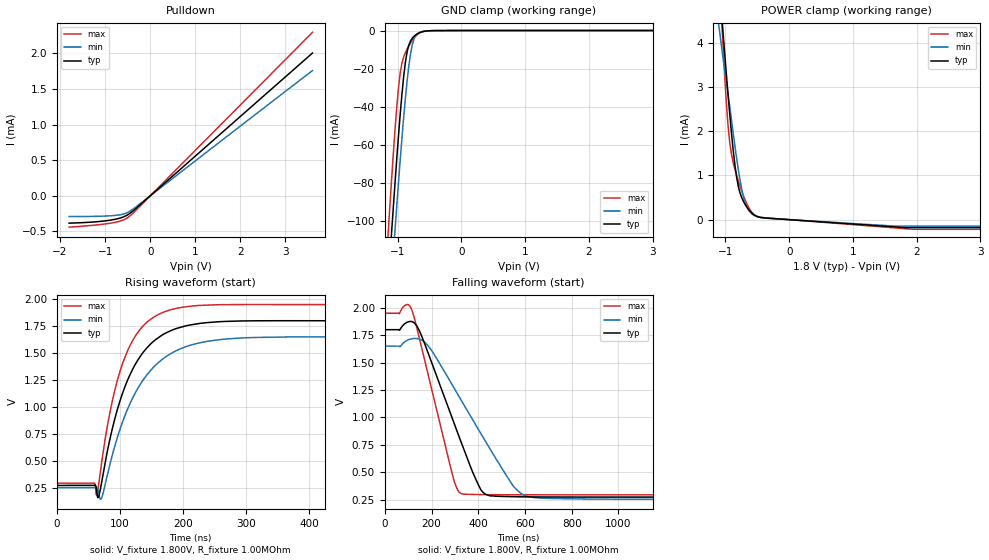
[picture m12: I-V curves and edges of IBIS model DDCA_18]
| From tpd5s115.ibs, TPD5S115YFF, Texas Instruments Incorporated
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[Model]   DDCA_18
Model_type   I/O_open_sink
Vinl = 800.000mV
Vinh = 2.000V
Vmeas = 1.500V
Rref = 1000000
Vref = 0V
Cref = 15pF
|   typ   min   max
|3-state
C_comp   1.1949pF   1.1694pF   1.2535pF
|pulldown
|C_comp   1.1949pF   1.1694pF   1.2499pF
[Voltage Range]   1.800V   1.650V   1.950V
|Junction temperature
[Temperature Range]   40.0   100.0   -40.0
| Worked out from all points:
|   slope of the pulldown table from 0 to 0.27 V, typ, clamps not added: 1.8 kohm
|   GND clamp passes 1 mA (typ) near -0.64 V on its own axis
|   POWER clamp passes 1 mA (typ) near -0.83 V on its own axis
|   falling waveform, V_fixture 1.800V, R_fixture 1.00MOhm: 20-80 % time 160ns typ, 234ns min, 113ns max; typ from 1.8 V to 0.274 V
|   rising waveform, V_fixture 1.800V, R_fixture 1.00MOhm: 20-80 % time 55.5ns typ, 66.4ns min, 45.9ns max; typ from 0.274 V to 1.8 V
|ambient temperature   25   85   -40|
[Pulldown]
|   Voltage   I(typ)   I(min)   I(max)
-1.8V     -382.5uA   -290uA     -439.1uA
-1.284V   -367.9uA   -288.3uA   -413.6uA
-904.5mV  -342.7uA   -280.5uA   -385.4uA
-633.2mV  -304.3uA   -260.8uA   -347.1uA
-470.4mV  -254uA     -222.9uA   -292.1uA
3.6V      2.002mA    1.756mA    2.293mA
[GND Clamp]
|   Voltage   I(typ)   I(min)   I(max)
-1.8V     -494.6mA   -503.4mA   -493.4mA
-1.149V   -134.2mA   -158mA     -107.5mA
-1.094V   -106.8mA   -131.2mA   -78.94mA
-1.04V    -80.42mA   -105.3mA   -52.46mA
-985.9mV  -55.68mA   -80.32mA   -30.36mA
-958.8mV  -44.25mA   -68.37mA   -22.43mA
-931.7mV  -33.73mA   -56.87mA   -17.18mA
-877.4mV  -16.86mA   -35.78mA   -11.65mA
-823.1mV  -7.647mA   -18.61mA   -8.038mA
-768.8mV  -4.04mA    -7.532mA   -5.134mA
-660.3mV  -1.221mA   -1.081mA   -1.428mA
3.6V      0A         0A         0A
[POWER Clamp]
|   Voltage   I(typ)   I(min)   I(max)
-1.8V     16.31mA    629.3uA    25.82mA
-1.637V   14.6mA     689.9uA    21.44mA
-1.61V    14.21mA    6.334mA    20.68mA
-1.094V   5.278mA    4.283mA    5.537mA
-1.04V    4.277mA    3.674mA    3.987mA
-958.8mV  2.821mA    2.825mA    2.114mA
-904.5mV  1.944mA    2.247mA    1.469mA
-823.1mV  944.1uA    1.373mA    995.8uA
-768.8mV  592.3uA    874.8uA    746.7uA
-687.4mV  333.7uA    370uA      432.5uA
-551.8mV  108.1uA    98.03uA    115.7uA
3.6V      -178.9uA   -145uA     -218.5uA
[Ramp]
R_load = 1.00MOhm
|   typ   min   max
dV/dt_r   915.721mV/55.495ns  837.785mV/66.402ns  993.306mV/45.871ns
dV/dt_f   915.721mV/160.189ns 837.785mV/233.595ns 993.306mV/112.779ns
[Falling Waveform]
V_fixture = 1.800V
V_fixture_min = 1.650V
V_fixture_max = 1.950V
R_fixture = 1.00MOhm
|   Time   V(typ)   V(min)   V(max)
0s        1.8V       1.65V      1.95V
114ns     1.874V     1.716V     1.989V
142ns     1.815V     1.718V     1.774V
187ns     1.579V     1.649V     1.373V
295ns     955mV      1.274V     432.7mV
325ns     784.5mV    1.164V     308.9mV
424ns     310.8mV    806.8mV    296.5mV
549ns     277.6mV    376.4mV    295mV
610ns     275.9mV    280.9mV    294.8mV
1.914us   273.8mV    253.7mV    294.5mV
[Rising Waveform]
V_fixture = 1.800V
V_fixture_min = 1.650V
V_fixture_max = 1.950V
R_fixture = 1.00MOhm
|   Time   V(typ)   V(min)   V(max)
0s        273.8mV    253.7mV    294.5mV
60ns      273.8mV    253.6mV    294.4mV
63ns      224.2mV    253.4mV    183.1mV
71ns      308.3mV    160.6mV    491.8mV
90ns      853.1mV    604mV      1.115V
113ns     1.265V     996.4mV    1.536V
149ns     1.588V     1.344V     1.817V
199ns     1.745V     1.548V     1.926V
346ns     1.801V     1.649V     1.95V
1.914us   1.8V       1.65V      1.95V
